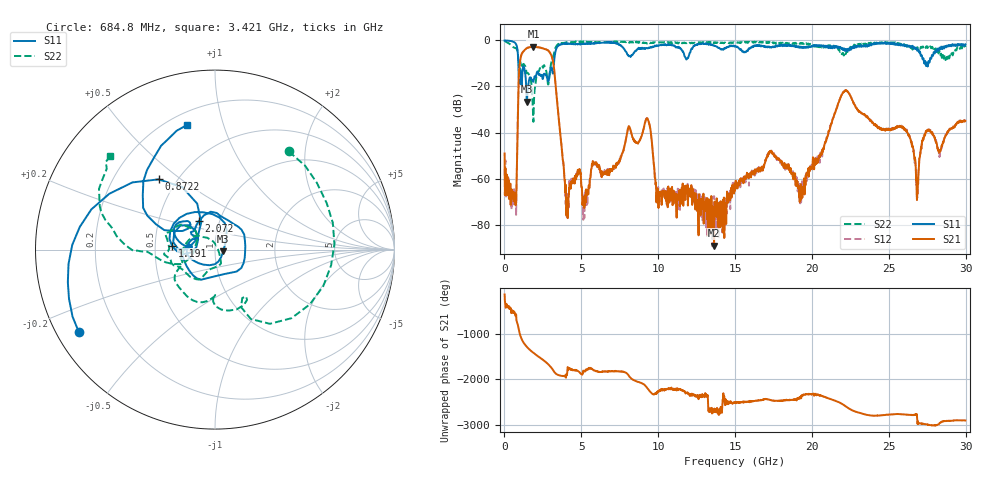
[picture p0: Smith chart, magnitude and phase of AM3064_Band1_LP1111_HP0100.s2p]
# Hz S DB R 50.0
!freq dBS11 angS11 dBS21 angS21 dBS12 angS12 dBS22 angS22
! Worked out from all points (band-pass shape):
!   1600 points, 10 MHz to 29.98 GHz, reference 50 ohm
!   highest |S21| = -2.71 dB at 1.884 GHz (marker M1); lowest = -89.0 dB at 13.64 GHz (marker M2)
!   |S21| within 3 dB of the highest: 1.134 GHz to 2.992 GHz (1.858 GHz wide, 90.1 % of centre)
!   lowest |S11| = -26.6 dB at 1.453 GHz (marker M3), VSWR 1.10, Z = 54.8 - j1.1 ohm
!   |S11| at or under -10 dB: 902.4 MHz to 3.22 GHz (2.318 GHz wide, 112 % of centre); 27.39383 GHz to 27.45833 GHz (64.49 MHz wide, 0.235 % of centre); 27.48917 GHz to 27.56368 GHz (74.51 MHz wide, 0.271 % of centre)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
!   |S22| runs from -35.3 to -0.2 dB; largest |S21 - S12| = 0.012
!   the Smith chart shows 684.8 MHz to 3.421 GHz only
!   S11 on the Smith chart (normalised r, x): 684.8 MHz: 0.06, -0.28; 872.2 MHz: 0.40, +0.42; 1.191 GHz: 0.61, +0.03; 2.072 GHz: 0.80, +0.26; 3.421 GHz: 0.27, +0.77
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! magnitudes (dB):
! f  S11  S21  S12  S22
! 10 MHz  0.0  -49.1  -55.7  -0.2
! 684.8 MHz  -1.0  -69.1  -67.9  -3.3
! 872.2 MHz  -6.0  -31.0  -30.9  -5.8
! 1.191 GHz  -12.4  -5.1  -5.0  -10.8
! 1.453 GHz  -26.6  -3.4  -3.3  -14.3
! 1.884 GHz  -17.8  -2.7  -2.8  -35.3
! 2.072 GHz  -14.8  -2.9  -2.8  -15.8
! 3.028 GHz  -11.8  -6.2  -6.1  -10.2
! 3.421 GHz  -2.9  -26.6  -26.4  -2.1
! 4.04 GHz  -1.5  -72.6  -66.4  -0.9
! 5.015 GHz  -1.6  -63.7  -64.2  -0.5
! 9.269 GHz  -3.4  -33.9  -33.6  -1.3
! 10 GHz  -2.2  -65.4  -63.6  -0.9
! 13.64 GHz  -2.3  -89.0  -67.5  -1.0
! 15 GHz  -2.7  -63.6  -64.4  -1.1
! 19.99 GHz  -2.8  -55.7  -54.8  -1.7
! 22.15 GHz  -4.5  -21.9  -21.7  -5.2
! 25 GHz  -1.0  -38.7  -38.1  -1.1
! 26.21 GHz  -2.2  -40.0  -40.1  -2.7
! 26.83 GHz  -4.2  -69.3  -63.1  -3.2
! 27.47 GHz  -9.6  -39.2  -39.0  -2.6
! 29.98 GHz  -1.7  -34.9  -35.1  -2.9
